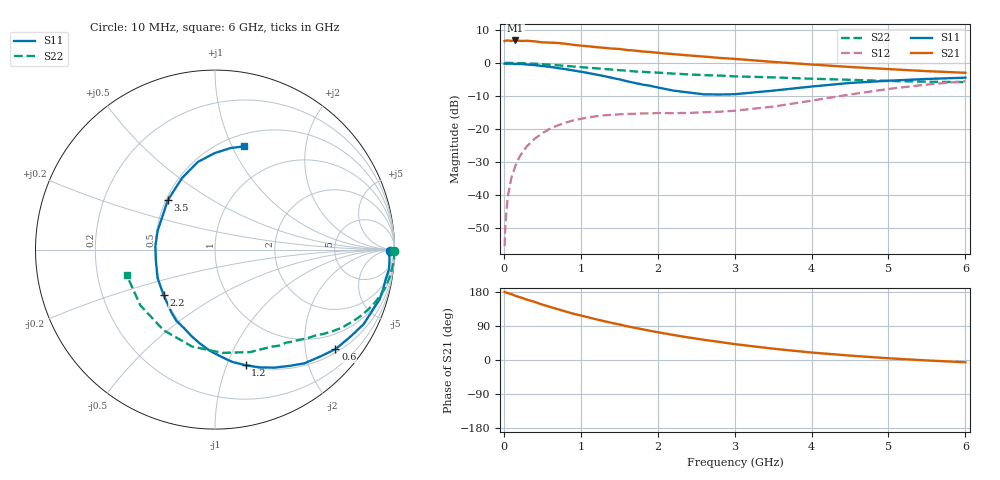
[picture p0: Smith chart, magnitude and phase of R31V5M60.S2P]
! SIEMENS Small Signal Semiconductors
! BFR181
! Si NPN RF Bipolar Junction Transistor in SOT23
! VCE = 1.5 V  IC = 0.6 mA
! Common Emitter S-Parameters:  May  1996
# GHz  S  MA  R  50
!  f  S11  S21  S12  S22
! GHz  MAG  ANG  MAG  ANG  MAG  ANG  MAG  ANG
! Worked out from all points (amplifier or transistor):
!   36 points, 10 MHz to 6 GHz, reference 50 ohm
!   highest |S21| = 6.8 dB at 150 MHz (marker M1)
!   |S21| within 3 dB of that: start of sweep to 1.663 GHz
!   unconditionally stable (mu >= 1): 2.225 GHz to 3.951 GHz
!   at 250 MHz: K = 0.12, MSG = 16.7 dB, |S12| = -26.7 dB
!   at 1.4 GHz: K = 0.65, MSG = 10.0 dB, |S12| = -15.7 dB
!   at 6 GHz: K = 0.92, MSG = 1.3 dB, |S12| = -5.5 dB
!   S11 on the Smith chart (normalised r, x): 10 MHz: 67, -28; 600 MHz: 0.58, -2.67; 1.2 GHz: 0.50, -1.17; 2.2 GHz: 0.50, -0.29; 3.5 GHz: 0.51, +0.33; 6 GHz: 0.62, +1.12
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0.01  0.975 -0.6  2.141 179.7  0.0017 89.2  0.9995 -0.4
0.02  0.9704 -1.3  2.165 178.6  0.0036 89.3  0.9991 -0.7
0.05  0.9741 -3.4  2.18 176.8  0.0094 86.5  0.9981 -1.6
0.1  0.9756 -6.5  2.148 173.7  0.0188 85.7  0.9987 -3.1
0.15  0.9648 -10.1  2.183 169.3  0.0278 83.0  0.9942 -4.9
0.2  0.9625 -13.1  2.149 166.2  0.0372 81.1  0.9914 -6.3
0.3  0.9443 -20.0  2.16 159.3  0.0549 76.3  0.9825 -9.6
0.4  0.9266 -26.6  2.117 153.4  0.0713 71.8  0.9721 -12.6
0.6  0.8706 -39.6  2.026 140.1  0.1013 63.9  0.9396 -18.2
0.8  0.8056 -51.9  1.946 128.2  0.125 56.3  0.9019 -23.3
1.1  0.7015 -69.3  1.782 112.5  0.15 47.5  0.8454 -29.7
1.2  0.6658 -75.2  1.728 107.3  0.1561 44.8  0.8284 -31.9
1.5  0.564 -93.0  1.625 93.8  0.1666 39.1  0.7757 -36.8
1.7  0.4985 -105.4  1.534 85.1  0.1697 36.9  0.7428 -39.7
2  0.4251 -125.0  1.419 73.3  0.1748 34.8  0.713 -43.9
2.2  0.3819 -138.7  1.358 66.2  0.174 35.0  0.6886 -46.9
2.6  0.3351 -169.5  1.246 53.3  0.1794 37.5  0.6528 -52.6
3  0.3363 162.1  1.15 41.9  0.1891 41.5  0.6261 -59.7
3.5  0.3808 133.7  1.035 29.9  0.2186 46.4  0.6036 -71.1
4.5  0.4976 101.1  0.867 11.6  0.3331 47.0  0.5549 -103.3
5.5  0.5719 81.4  0.75 -1.2  0.4705 34.4  0.5192 -143.2
6  0.598 74.2  0.709 -6.0  0.5283 26.1  0.512 -163.7
